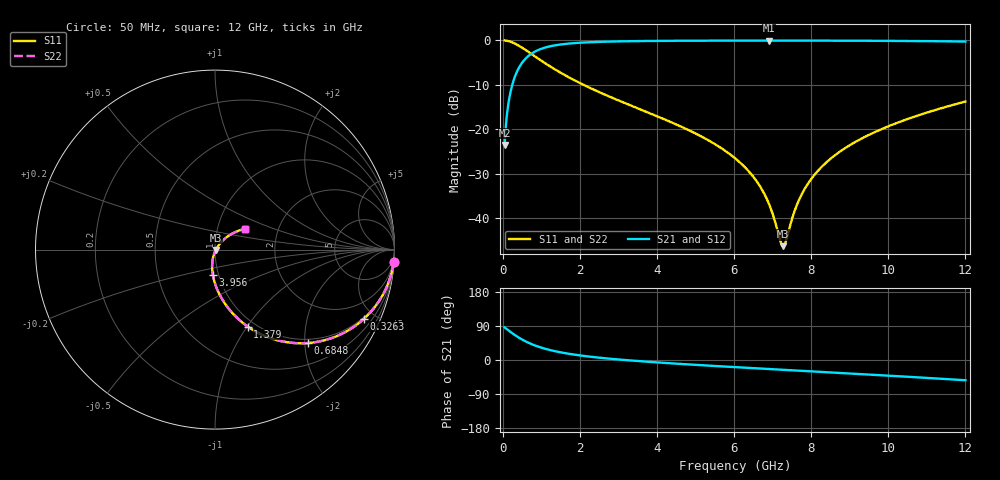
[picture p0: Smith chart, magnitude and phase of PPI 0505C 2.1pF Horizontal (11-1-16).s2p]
# MHz S MA R 50
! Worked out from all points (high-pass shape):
!   1601 points, 50 MHz to 12 GHz, reference 50 ohm
!   highest |S21| = -0.05 dB at 6.899 GHz (marker M1); lowest = -23.5 dB at 50 MHz (marker M2)
!   |S21| within 3 dB of the highest: 736.2 MHz to end of sweep
!   lowest |S11| = -46.2 dB at 7.272 GHz (marker M3), VSWR 1.01, Z = 50.4 - j0.225 ohm
!   |S11| at or under -10 dB: 2.1 GHz to end of sweep
!   |S22| runs from -46.2 to 0.0 dB; largest |S21 - S12| = 0
!   S11 on the Smith chart (normalised r, x): 50 MHz: 1, -28; 326.3 MHz: 0.91, -4.36; 684.8 MHz: 0.92, -2.07; 1.379 GHz: 0.92, -1.00; 3.956 GHz: 0.94, -0.27; 12 GHz: 1.36, +0.33
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50  0.9978 -4.0  0.06688 86.0  0.06688 86.0  0.9978 -4.0
176.9688  0.9729 -14.0  0.2309 76.0  0.2309 76.0  0.9729 -14.0
326.3438  0.9157 -24.8  0.4012 65.1  0.4012 65.1  0.9157 -24.8
490.6562  0.8342 -35.2  0.5504 54.8  0.5504 54.8  0.8342 -35.2
684.8438  0.7339 -45.2  0.6779 44.7  0.6779 44.7  0.7339 -45.2
1006  0.5897 -57.3  0.8059 32.5  0.8059 32.5  0.5897 -57.3
1379.438  0.4656 -67.0  0.8829 22.8  0.8829 22.8  0.4656 -67.0
2044.156  0.325 -78.0  0.9431 11.6  0.9431 11.6  0.325 -78.0
3956.156  0.1434 -94.6  0.986 -6.0  0.986 -6.0  0.1434 -94.6
4038.312  0.1386 -95.1  0.9866 -6.6  0.9866 -6.6  0.1386 -95.1
5225.844  0.08015 -101.3  0.9925 -14.2  0.9925 -14.2  0.08015 -101.3
6025  0.04753 -103.6  0.9942 -18.8  0.9942 -18.8  0.04753 -103.6
6540.344  0.02791 -102.4  0.9947 -21.8  0.9947 -21.8  0.02791 -102.4
6898.844  0.01482 -95.2  0.9948 -23.8  0.9948 -23.8  0.01482 -95.2
7197.594  0.005651 -56.3  0.9947 -25.4  0.9947 -25.4  0.005651 -56.3
7272.281  0.004888 -27.2  0.9947 -25.8  0.9947 -25.8  0.004888 -27.2
7346.969  0.005602 2.3  0.9946 -26.3  0.9946 -26.3  0.005602 2.3
7668.125  0.01555 42.9  0.9943 -28.1  0.9943 -28.1  0.01555 42.9
8019.156  0.02843 49.3  0.9938 -30.0  0.9938 -30.0  0.02843 49.3
8803.375  0.05862 50.0  0.9921 -34.4  0.9921 -34.4  0.05862 50.0
10013.31  0.109 45.3  0.987 -41.3  0.987 -41.3  0.109 45.3
12000  0.2057 34.4  0.9701 -53.4  0.9701 -53.4  0.2057 34.4
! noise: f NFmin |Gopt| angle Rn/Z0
50  0.0008124  0.9466  1.816  0.00341
1372  0.005591  0.7576  6.155  0.004654
2701  0.008932  0.7094  10.61  0.005998
4031  0.01192  0.6818  15.12  0.00713
5360  0.01477  0.6645  19.58  0.008203
6682  0.01758  0.6543  23.94  0.009287
8012  0.02047  0.6492  28.23  0.01045
9341  0.02348  0.6486  32.41  0.01174
1.067e+04  0.02669  0.6517  36.48  0.01321
1.2e+04  0.03018  0.6581  40.43  0.01493
